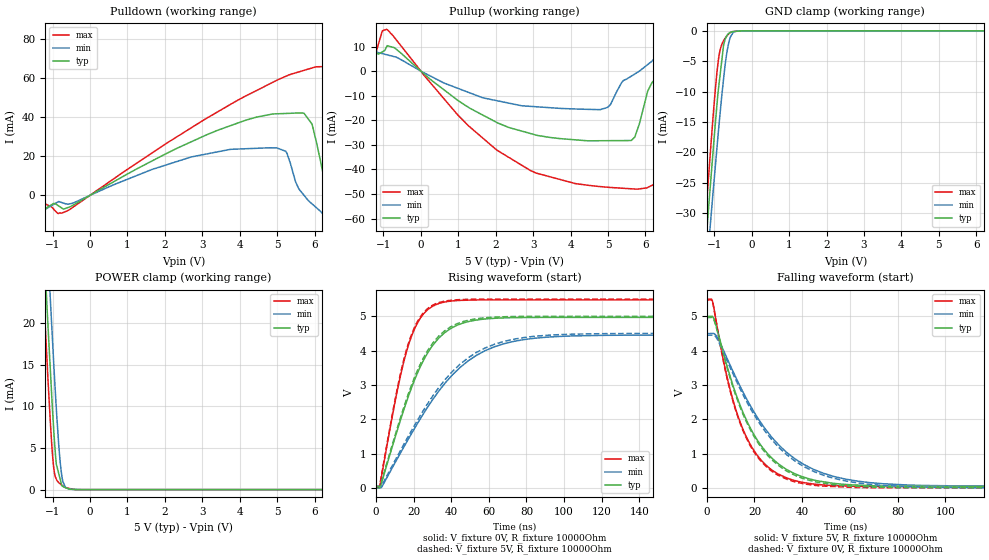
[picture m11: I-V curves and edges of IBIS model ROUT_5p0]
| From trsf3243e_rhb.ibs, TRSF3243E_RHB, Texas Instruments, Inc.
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[Model]   ROUT_5p0
Model_type   3-state
Polarity   Non-Inverting
Vmeas = 2.5
Vref = 0
Cref = 150pF
Rref = 3000
|variable   typ   min   max
C_comp   1.38pF   1.30pF   1.43pF
|C_pullup   1.31pF   1.23pF   1.37pF
|C_pulldown   1.78pF   1.74pF   1.85pF
[Voltage Range]   5   4.5   5.5
[Temperature Range]   27   110   -40
[Pullup Reference]   5   4.5   5.5
[Pulldown Reference]   0   0   0
[Power Clamp Reference]   5   4.5   5.5
[GND Clamp Reference]   0   0   0
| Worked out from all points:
|   slope of the pulldown table from 0 to 0.75 V, typ, clamps not added: 91.3 ohm
|   slope of the pullup table from 0 to 0.75 V, typ, clamps not added: 81.9 ohm
|   GND clamp passes 1 mA (typ) near -0.68 V on its own axis
|   POWER clamp passes 1 mA (typ) near -0.78 V on its own axis
|   falling waveform, V_fixture 5V, R_fixture 10000Ohm: 20-80 % time 18.4ns typ, 25.7ns min, 14.3ns max; typ from 5 V to 0.039 V
|   rising waveform, V_fixture 0V, R_fixture 10000Ohm: 20-80 % time 20.4ns typ, 34.1ns min, 13.2ns max; typ from 0 V to 4.97 V
|   rising waveform, V_fixture 5V, R_fixture 10000Ohm: 20-80 % time 20.1ns typ, 33.3ns min, 13.1ns max; typ from 0.039 V to 5 V
|   falling waveform, V_fixture 0V, R_fixture 10000Ohm: 20-80 % time 18.3ns typ, 25.4ns min, 14.3ns max; typ from 4.97 V to 0 V
[Pulldown]
|   Voltage   I(typ)   I(min)   I(max)
-5V       -780.8uA   -278.4uA   -898.2uA
-764.5mV  -6.348mA   -3.623mA   -9.147mA
4.882V    41.67mA    24.34mA    57.85mA
5.716V    42.05mA    48.26uA    64mA
6.228V    11.15mA    -9.654mA   65.9mA
6.544V    -20.3uA    -13.84mA   58.36mA
7.073V    -13.01mA   -14.06mA   8.908mA
7.792V    -13.95mA   -14.24mA   -12.54mA
9.735V    -13.05mA   -13.19mA   -14.43mA
9.886V    -10.99mA   -9.056mA   -5.798mA
9.915V    91.58mA    -8.283mA   81.7mA
10V       399.8mA    457.1mA    344.6mA
[GND Clamp]
|   Voltage   I(typ)   I(min)   I(max)
-5V       -355.6mA   -336.7mA   -374.9mA
-1.338V   -44.36mA   -49.37mA   -40.19mA
-1.205V   -33.57mA   -39.45mA   -28.67mA
-1.163V   -30.18mA   -36.27mA   -25.03mA
-1.135V   -27.99mA   -34.25mA   -22.74mA
-1.089V   -24.36mA   -30.81mA   -18.83mA
-973.6mV  -15.53mA   -22.56mA   -9.873mA
-867.4mV  -8.559mA   -15.17mA   -3.914mA
-750.6mV  -2.375mA   -7.945mA   -1.647mA
-658.6mV  -799.2uA   -3.415mA   -780.7uA
-521.1mV  -136.1uA   -548.3uA   -156.3uA
10V       0A         0A         0A
[Pullup]
|   Voltage   I(typ)   I(min)   I(max)
-5V       98.14uA    69.08uA    126.7uA
-4.742V   15mA       14.94mA    15.05mA
-911.9mV  9.999mA    6.652mA    17.02mA
2.029V    -20.9mA    -12.03mA   -32.14mA
5.777V    -24.16mA   -600.8uA   -48.04mA
6.193V    -4.317mA   4.357mA    -46.36mA
6.853V    2.92mA     8.214mA    -7.749mA
7.792V    8.278mA    8.328mA    8.582mA
9.735V    7.295mA    7.355mA    9.879mA
9.885V    5.533mA    4.087mA    6.708mA
9.915V    -85.71mA   3.431mA    -81.8mA
10V       -359.8mA   -379.7mA   -332.8mA
[POWER Clamp]
|   Voltage   I(typ)   I(min)   I(max)
-5V       399.5mA    407.3mA    393.9mA
-1.338V   39.38mA    48.14mA    32.77mA
-1.205V   27.08mA    35.95mA    20.57mA
-1.157V   22.77mA    31.52mA    16.31mA
-1.082V   16.27mA    24.77mA    9.909mA
-1.06V    14.41mA    22.89mA    8.13mA
-973.6mV  7.547mA    15.58mA    2.804mA
-900.9mV  3.072mA    9.867mA    1.276mA
-815.6mV  1.585mA    4.271mA    761.5uA
-759.7mV  610.8uA    1.847mA    554.6uA
-582.8mV  106.4uA    113.1uA    169.6uA
10V       0A         0A         0A
[Ramp]
R_load = 10000
|   typ   min   max
dV/dt_r   2.98109/2.04131e-08   2.67144/3.41326e-08   3.2869/1.32517e-08
dV/dt_f   2.97654/1.8391e-08   2.67255/2.57068e-08   3.27911/1.43282e-08
[Falling Waveform]
V_fixture = 5V
V_fixture_min = 4.5V
V_fixture_max = 5.5V
R_fixture = 10000Ohm
C_fixture = 0F
|   Time   V(typ)   V(min)   V(max)
0s        5V         4.5V       5.5V
2.43ns    4.997V     4.503V     5.439V
8.848ns   3.473V     3.727V     3.136V
12.4ns    2.703V     3.192V     2.237V
16.22ns   2.042V     2.658V     1.543V
23.24ns   1.19V      1.846V     773.4mV
33.78ns   525.1mV    1.019V     281.3mV
49.01ns   177.2mV    422.9mV    84.63mV
73.58ns   55.02mV    121.5mV    38.23mV
200ns     39.1mV     45.76mV    34.81mV
[Rising Waveform]
V_fixture = 0V
V_fixture_min = 0V
V_fixture_max = 0V
R_fixture = 10000Ohm
C_fixture = 0F
|   Time   V(typ)   V(min)   V(max)
0s        -139.6nV   -88.58nV   -98.3nV
1.973ns   -908.4uV   -22.57uV   26.62mV
11.12ns   1.635V     826.1mV    2.769V
17.61ns   2.721V     1.457V     4.216V
23.24ns   3.49V      1.981V     4.917V
31.7ns    4.255V     2.69V      5.336V
39.76ns   4.646V     3.238V     5.442V
49.01ns   4.844V     3.701V     5.47V
73.58ns   4.96V      4.273V     5.478V
200ns     4.968V     4.452V     5.478V
[Rising Waveform]
V_fixture = 5V
V_fixture_min = 4.5V
V_fixture_max = 5.5V
R_fixture = 10000Ohm
C_fixture = 0F
|   Time   V(typ)   V(min)   V(max)
0s        39.1mV     45.83mV    34.81mV
1.973ns   38.21mV    45.8mV     61.49mV
11.12ns   1.699V     895.1mV    2.828V
17.61ns   2.796V     1.543V     4.27V
23.24ns   3.564V     2.077V     4.959V
29.68ns   4.177V     2.635V     5.31V
39.76ns   4.695V     3.338V     5.466V
49.01ns   4.884V     3.791V     5.494V
73.58ns   4.993V     4.336V     5.5V
200ns     5V         4.5V       5.5V
[Falling Waveform]
|Gnd
V_fixture = 0V
V_fixture_min = 0V
V_fixture_max = 0V
R_fixture = 10000Ohm
C_fixture = 0F
|   Time   V(typ)   V(min)   V(max)
0s        4.968V     4.452V     5.478V
2.405ns   4.966V     4.454V     5.421V
8.848ns   3.426V     3.662V     3.101V
12.4ns    2.654V     3.121V     2.2V
16.22ns   1.992V     2.583V     1.505V
23.24ns   1.142V     1.771V     736.3mV
33.78ns   480.8mV    951.5mV    245.3mV
49.01ns   136.1mV    366.1mV    52.06mV
73.58ns   15.59mV    72.69mV    3.382mV
200ns     -5.346uV   -64.64uV   4.327uV
